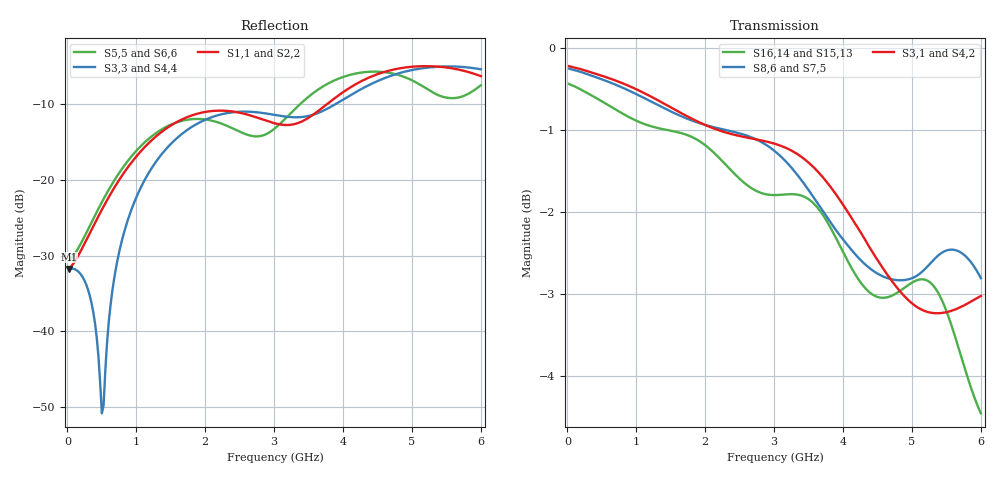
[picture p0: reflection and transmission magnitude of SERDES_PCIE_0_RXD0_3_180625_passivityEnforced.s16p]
! RTG4 CQ352 S-parameter file
! Microsemi Corporation (c) 2019
!Initial ver: Feb 12, 2019
! Port::NET_NAME::S-parameter ports::PORT SIDE
! Port1::SERDES_PCIE_0_RXD0_N::1::DIE
! Port2::SERDES_PCIE_0_RXD0_P::2::DIE
! Port3::SERDES_PCIE_0_RXD0_N::3::Lead
! Port4::SERDES_PCIE_0_RXD0_P::4::Lead
! Port5::SERDES_PCIE_0_RXD1_N::5::DIE
! Port6::SERDES_PCIE_0_RXD1_P::6::DIE
! Port7::SERDES_PCIE_0_RXD1_N::7::Lead
! Port8::SERDES_PCIE_0_RXD1_P::8::Lead
! Port9::SERDES_PCIE_0_RXD2_N::9::DIE
! Port10::SERDES_PCIE_0_RXD2_P::10::DIE
! Port11::SERDES_PCIE_0_RXD2_N::11::Lead
! Port12::SERDES_PCIE_0_RXD2_P::12::Lead
! Port13::SERDES_PCIE_0_RXD3_N::13::DIE
! Port14::SERDES_PCIE_0_RXD3_P::14::DIE
! Port15::SERDES_PCIE_0_RXD3_N::15::Lead
! Port16::SERDES_PCIE_0_RXD3_P::16::Lead
!PowerSI Version: 17.0.2.03131.86335  002
!Computer Host Name: W764D-PINDIS
!TouchstoneFormatFlag = 1
! GNDNET
! NETSLIST
!User Comments:
!  Touchstone file from project YBDH07-1_op7_160920_RXD_0-3
!  Exported from HFSS 2016.2.0
!  Terminal data exported
!  Port[1] = FC_SERDES_PCIE_0_RXD0_N_T1
!  Port[2] = FC_SERDES_PCIE_0_RXD0_P_T1
!  Port[3] = LEAD_9_32_T1
!  Port[4] = LEAD_9_33_T1
!  Port[5] = FC_SERDES_PCIE_0_RXD1_N_T1
!  Port[6] = FC_SERDES_PCIE_0_RXD1_P_T1
!  Port[7] = LEAD_9_24_T1
!  Port[8] = LEAD_9_25_T1
!  Port[9] = FC_SERDES_PCIE_0_RXD2_N_T1
!  Port[10] = FC_SERDES_PCIE_0_RXD2_P_T1
!  Port[11] = LEAD_9_2_T1
!  Port[12] = LEAD_9_3_T1
!  Port[13] = FC_SERDES_PCIE_0_RXD3_N_T1
!  Port[14] = FC_SERDES_PCIE_0_RXD3_P_T1
!  Port[15] = LEAD_2_T1
!  Port[16] = LEAD_10_T1
#	Hz	S	DB	R	50
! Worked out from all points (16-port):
!   240 points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, 25 MHz to 6 GHz, reference 50 ohm
!   strongest paths, dB at 25 MHz, 1.525 GHz, 3.025 GHz, 4.525 GHz, 6 GHz:
!     S3,1: -0.2, -0.7, -1.2, -2.6, -3.0
!     S4,2: -0.2, -0.7, -1.2, -2.7, -3.1
!     S8,6: -0.3, -0.8, -1.3, -2.8, -2.8
!     S7,5: -0.3, -0.8, -1.3, -2.9, -2.8
!     S16,14: -0.4, -1.0, -1.8, -3.0, -4.4
!     S15,13: -0.4, -1.0, -1.8, -3.1, -4.6
!   lowest |S11| = -31.8 dB at 25 MHz (marker M1), VSWR 1.05, Z = 52.6 + j0.0763 ohm
!   |S11| at or under -10 dB: start of sweep to 3.772 GHz
